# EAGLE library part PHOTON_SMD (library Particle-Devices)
Photon (without headers) - designed to be surface mounted with 7 extra exposed pads on the bottom of the board which include, 3 RGB LED outputs, /SETUP, EN (3.3V SMPS enable input), USB D+ and USB D-.
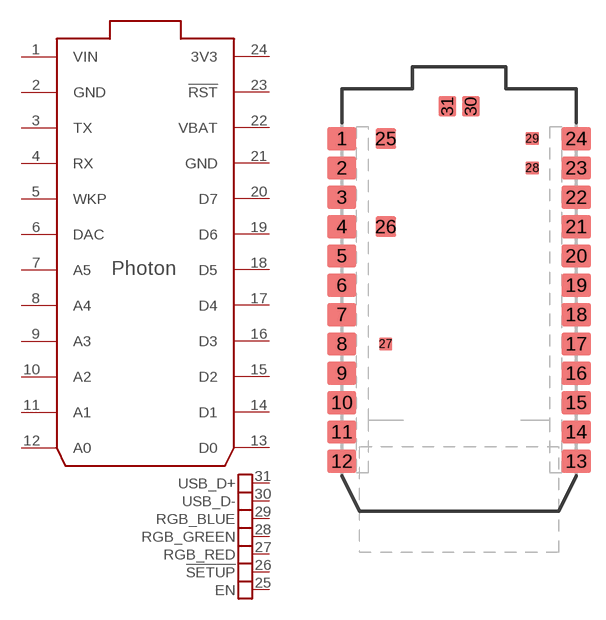
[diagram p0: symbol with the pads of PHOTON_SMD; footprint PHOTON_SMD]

Designator prefix -; gates G$1=PHOTON G$2=PHOTON_PADS

## PHOTON_SMD  [PHOTON_SMD]
1  G$1:VIN  pwr
2  G$1:GND  pwr
3  G$1:TX
4  G$1:RX
5  G$1:WKP
6  G$1:DAC
7  G$1:A5
8  G$1:A4
9  G$1:A3
10  G$1:A2
11  G$1:A1
12  G$1:A0
13  G$1:D0
14  G$1:D1
15  G$1:D2
16  G$1:D3
17  G$1:D4
18  G$1:D5
19  G$1:D6
20  G$1:D7
21  G$1:GND  pwr
22  G$1:VBAT  pwr
23  G$1:!RST
24  G$1:3V3  pwr
25  G$2:EN
26  G$2:!SETUP
27  G$2:RGB_RED
28  G$2:RGB_GREEN
29  G$2:RGB_BLUE
30  G$2:USB_D-
31  G$2:USB_D+

## Footprint PHOTON_SMD (pad centres in mm)
smd 2.54 x 2.032: 1 0,32.258; 2 0,29.718; 3 0,27.178; 4 0,24.638; 5 0,22.098; 6 0,19.558; 7 0,17.018; 8 0,14.478; 9 0,11.938; 10 0,9.398; 11 0,6.858; 12 0,4.318; 13 20.32,4.318; 14 20.32,6.858; 15 20.32,9.398; 16 20.32,11.938; 17 20.32,14.478; 18 20.32,17.018; 19 20.32,19.558; 20 20.32,22.098; 21 20.32,24.638; 22 20.32,27.178; 23 20.32,29.718; 24 20.32,32.258
smd 1.778 x 1.778: 25 3.81,32.258; 26 3.81,24.638
smd 1.143 x 1.143: 27 3.81,14.478; 28 16.51,29.718; 29 16.51,32.258
smd 1.524 x 1.778: 30 11.176,35.052; 31 9.144,35.052

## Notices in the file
Licensing: Designed by Particle.
